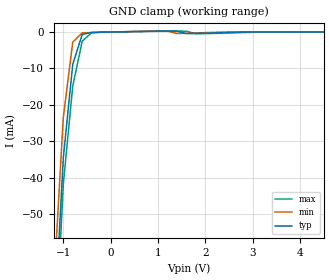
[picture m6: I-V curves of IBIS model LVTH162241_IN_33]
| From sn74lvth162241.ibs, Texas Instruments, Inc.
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|   Model LVTH162241 Input_IN_33
[Model]   LVTH162241_IN_33
Model_type  Input
Polarity   Non-Inverting
Vinl = 0.8V
Vinh = 2.0V
| variable   typ   min   max
C_comp   4pf   NA   NA
[Temperature Range]   40   -25   100
| Ambient temperature   25   -40   85
[Voltage range]   3.3   3.0   3.6
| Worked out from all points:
|   GND clamp passes 1 mA (typ) near -0.61 V on its own axis
[GND Clamp]
|   Voltage   I(typ)   I(min)   I(max)
-5V       -1.689A    -1.778A    -1.539A
-1.2V     -83.34mA   -69.28mA   -94.22mA
-1V       -34.56mA   -23.46mA   -41.78mA
-800mV    -8.857mA   -2.738mA   -14.81mA
-600mV    -634.2uA   -232.4uA   -2.519mA
-400mV    -117.8uA   -132.5uA   -148.4uA
-200mV    -57.39uA   -65.17uA   -51.99uA
1.2V      257.5uA    271.5uA    244.4uA
1.4V      244.8uA    -404.1uA   254.4uA
1.6V      -440.6uA   -341.7uA   225.6uA
1.8V      -387.1uA   -260.7uA   -475.1uA
5V        -363pA     586.3pA    749.5pA
